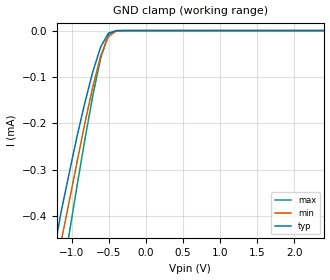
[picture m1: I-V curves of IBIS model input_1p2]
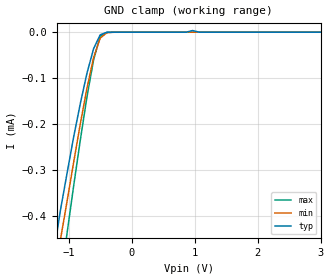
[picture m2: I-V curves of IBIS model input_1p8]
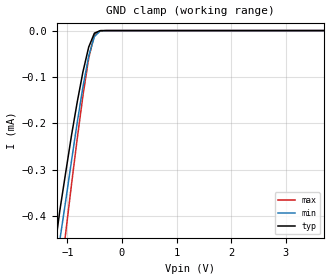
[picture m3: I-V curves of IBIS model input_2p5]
| Texas Instruments Incorporated
| SN74LXC1T45 Single-Channel Dual Supply Voltage Translator
| with 3-State outputs and Schmitt-trigger Inputs
[IBIS Ver]   4.1
[File name]   sn74lxc1t45.ibs
[File Rev]   1.0
[Date]   04/24/2019
[Source]
| Texas Instruments Incorporated.
| Analog-eLab Design Center, HPA
| 12500 TI Blvd
| Dallas, TX -75243
[Notes]   Revision History:
| Rev 1.0: 09/01/2020
| - Initial version of the model
| - Model generated from simulations in SPECTRE
| - C_comp although listed in numerical order of value are
|   obtained from varying PVT conditions. For PVT conditions for
|   each specific value refer the buffer description under
|   respective [Model]. IBIS model user is responsible for using
|   appropriate C_comp to simulate for Signal Integrity.
| - Warnings regarding combined Non-monotonicity of various models have been
|   reviewd and considered minor and can be ignored.
| - Model names with a trailing _2p5 contain the model for 2.5V operation.
[Disclaimer]
| This model is designed as an aid for customers of Texas Instruments.
| TI and its licensors and suppliers make no warranties, either expressed
| or implied, with respect to this  model, including the warranties of
| merchantability or fitness for a particular purpose. The model is
| provided solely on an "as is" basis. The entire risk as to its quality
| and performance is with the customer.
| This model is subject to change without notice. Texas Instruments
| Incorporated is not responsible for updating this model.
[Copyright]
 (C) Copyright 2020 Texas Instruments Incorporated.All rights reserved.
|Component SN74LXC1T45DBV 6-pin SOT - DBV package
|  Part # SN74LXC1T45DBV
[Component]   SN74LXC1T45DBV
[Manufacturer]  TI
[Package]   |6 SOT - DBV package
|   typ   min   max
R_pkg   0.05   0.04   0.06
L_pkg   1.0nH   0.8nH   1.2nH
C_pkg   0.2pF   0.16pF   0.24pF
[Pin]  signal_name model_name   R_pin   L_pin   C_pin
1   VCCA   power   NA   NA   NA
2   GND   gnd   NA   NA   NA
3   A   I/O   NA   NA   NA
4   B   I/O   NA   NA   NA
5   DIR   input   NA   NA   NA
6   VCCB   power   NA   NA   NA
|Component SN74LXC1T45DRL 6-pin SOT - DRL package
|  Part # SN74LXC1T45DRL
[Component]   SN74LXC1T45DRL
[Manufacturer]  TI
[Package]   |6 SOT - DRL package
|   typ   min   max
R_pkg   0.05   0.04   0.06
L_pkg   1.0nH   0.8nH   1.2nH
C_pkg   0.2pF   0.16pF   0.24pF
[Pin]  signal_name model_name   R_pin   L_pin   C_pin
1   VCCA   power   NA   NA   NA
2   GND   gnd   NA   NA   NA
3   A   I/O   NA   NA   NA
4   B   I/O   NA   NA   NA
5   DIR   input   NA   NA   NA
6   VCCB   power   NA   NA   NA
|Component SN74LXC1T45DCK 6-pin SOT - DCK package
|  Part # SN74LXC1T45DCK
[Component]   SN74LXC1T45DCK
[Manufacturer]  TI
[Package]   |6 SOT - DCK package
|   typ   min   max
R_pkg   0.05   0.04   0.06
L_pkg   1.0nH   0.8nH   1.2nH
C_pkg   0.2pF   0.16pF   0.24pF
[Pin]  signal_name model_name   R_pin   L_pin   C_pin
1   VCCA   power   NA   NA   NA
2   GND   gnd   NA   NA   NA
3   A   I/O   NA   NA   NA
4   B   I/O   NA   NA   NA
5   DIR   input   NA   NA   NA
6   VCCB   power   NA   NA   NA
|Component SN74LXC1T45DRY 6-pin SON - DRY package
|  Part # SN74LXC1T45DRY
[Component]   SN74LXC1T45DRY
[Manufacturer]  TI
[Package]   |6 SON - DRY package
|   typ   min   max
R_pkg   0.05   0.04   0.06
L_pkg   1.0nH   0.8nH   1.2nH
C_pkg   0.2pF   0.16pF   0.24pF
[Pin]  signal_name model_name   R_pin   L_pin   C_pin
1   VCCA   power   NA   NA   NA
2   GND   gnd   NA   NA   NA
3   A   I/O   NA   NA   NA
4   B   I/O   NA   NA   NA
5   DIR   input   NA   NA   NA
6   VCCB   power   NA   NA   NA
|Component SN74LXC1T45DTQ 6-pin X2SON - DTQ package
|  Part # SN74LXC1T45DTQ
[Component]   SN74LXC1T45DTQ
[Manufacturer]  TI
[Package]   |6 X2SON - DTQ package
|   typ   min   max
R_pkg   0.05   0.04   0.06
L_pkg   1.0nH   0.8nH   1.2nH
C_pkg   0.2pF   0.16pF   0.24pF
[Pin]  signal_name model_name   R_pin   L_pin   C_pin
1   VCCA   power   NA   NA   NA
2   GND   gnd   NA   NA   NA
3   A   I/O   NA   NA   NA
4   B   I/O   NA   NA   NA
5   DIR   input   NA   NA   NA
6   VCCB   power   NA   NA   NA
|   Model Selectors
[Model Selector] input
input_1p2   1.2V   digital input
input_1p8   1.8V   digital input
input_2p5   2.5V   digital input
input_3p3   3.3V   digital input
input_5p0   5.0V   digital input
[Model Selector] I/O
io_1p2   1.2V   Vcc
io_1p8   1.8V   Vcc
io_2p5   2.5V   Vcc
io_3p3   3.3V   Vcc
io_5p0   5.0V   Vcc
| Models and submodels in the file (10): input_1p2 (Input), input_1p8 (Input), input_2p5 (Input), input_3p3 (Input), input_5p0 (Input), io_1p2 (I/O), io_1p8 (I/O), io_2p5 (I/O), io_3p3 (I/O), io_5p0 (I/O)
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|   input_1p2 Model
[Model]   input_1p2
Model_type   Input
Vinl = 0.2
Vinh = 0.9
|   typ   min   max
C_comp   0.119pF   0.105pF   0.126pF
[Voltage Range]   1.2   1.08   1.32
|Junction Temperature
[Temperature Range]   25   125   -40
[GND Clamp Reference]   0   0   0
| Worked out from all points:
|   GND clamp passes 1 mA (typ) near -1.81 V on its own axis
[GND Clamp]
|   Voltage   I(typ)   I(min)   I(max)
-2.5V     -1.66mA    -1.64mA    -2.09mA
-1.24V    -478uA     -541uA     -650uA
-1.14V    -389uA     -453uA     -542uA
-1.03V    -305uA     -366uA     -435uA
-925mV    -226uA     -281uA     -332uA
-820mV    -154uA     -198uA     -233uA
-715mV    -88.7uA    -121uA     -140uA
-610mV    -35.6uA    -54.9uA    -59.7uA
-505mV    -5.5uA     -12.7uA    -8.49uA
-400mV    -210nA     -1.13uA    -141nA
8V        3.62nA     3.43nA     4.23nA
|   input_1p8 Model
[Model]   input_1p8
Model_type   Input
Vinl = 0.7
Vinh = 1.1
|   typ   min   max
C_comp   3.13pF   2.65pF   3.82pF
| Where Nom  PVT is Nominal Process, 2.25V, 27C
|   Fast PVT is Strong Process,  2.50V, -55C
|   Slow PVT is Weak Process,   2.0V, 150C
[Voltage Range]   1.8   1.62   1.98
|Junction Temperature
[Temperature Range]   25   125   -40
[GND Clamp Reference]   0   0   0
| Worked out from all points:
|   GND clamp passes 1 mA (typ) near -1.81 V on its own axis
[GND Clamp]
|   Voltage   I(typ)   I(min)   I(max)
-2.5V     -1.66mA    -1.64mA    -2.09mA
-1.24V    -478uA     -541uA     -650uA
-1.14V    -389uA     -453uA     -542uA
-1.03V    -305uA     -366uA     -435uA
-820mV    -154uA     -198uA     -233uA
-715mV    -88.7uA    -121uA     -140uA
-610mV    -35.6uA    -54.9uA    -59.7uA
-505mV    -5.5uA     -12.7uA    -8.49uA
-400mV    -210nA     -1.13uA    -141nA
965mV     3.74uA     3.02nA     4.93nA
1.07V     3.25nA     2.95nA     3.92nA
8V        3.62nA     3.43nA     4.23nA
|   input_2p5 Model
[Model]   input_2p5
Model_type   Input
Vinl = 1.0
Vinh = 1.4
|   typ   min   max
C_comp   3.03pF   2.54pF   3.83pF
| Where Nom  PVT is Nominal Process, 2.25V, 27C
|   Fast PVT is Strong Process,  2.50V, -55C
|   Slow PVT is Weak Process,   2.0V, 150C
[Voltage Range]   2.5   2.25   2.75
|Junction Temperature
[Temperature Range]   25   125   -40
[GND Clamp Reference]   0   0   0
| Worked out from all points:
|   GND clamp passes 1 mA (typ) near -1.81 V on its own axis
[GND Clamp]
|   Voltage   I(typ)   I(min)   I(max)
-2.5V     -1.66mA    -1.64mA    -2.09mA
-1.24V    -478uA     -541uA     -650uA
-1.14V    -389uA     -453uA     -542uA
-1.03V    -305uA     -366uA     -435uA
-925mV    -226uA     -281uA     -332uA
-820mV    -154uA     -198uA     -233uA
-715mV    -88.7uA    -121uA     -140uA
-610mV    -35.6uA    -54.9uA    -59.7uA
-505mV    -5.5uA     -12.7uA    -8.49uA
-400mV    -210nA     -1.14uA    -141nA
8V        3.62nA     3.43nA     4.23nA
